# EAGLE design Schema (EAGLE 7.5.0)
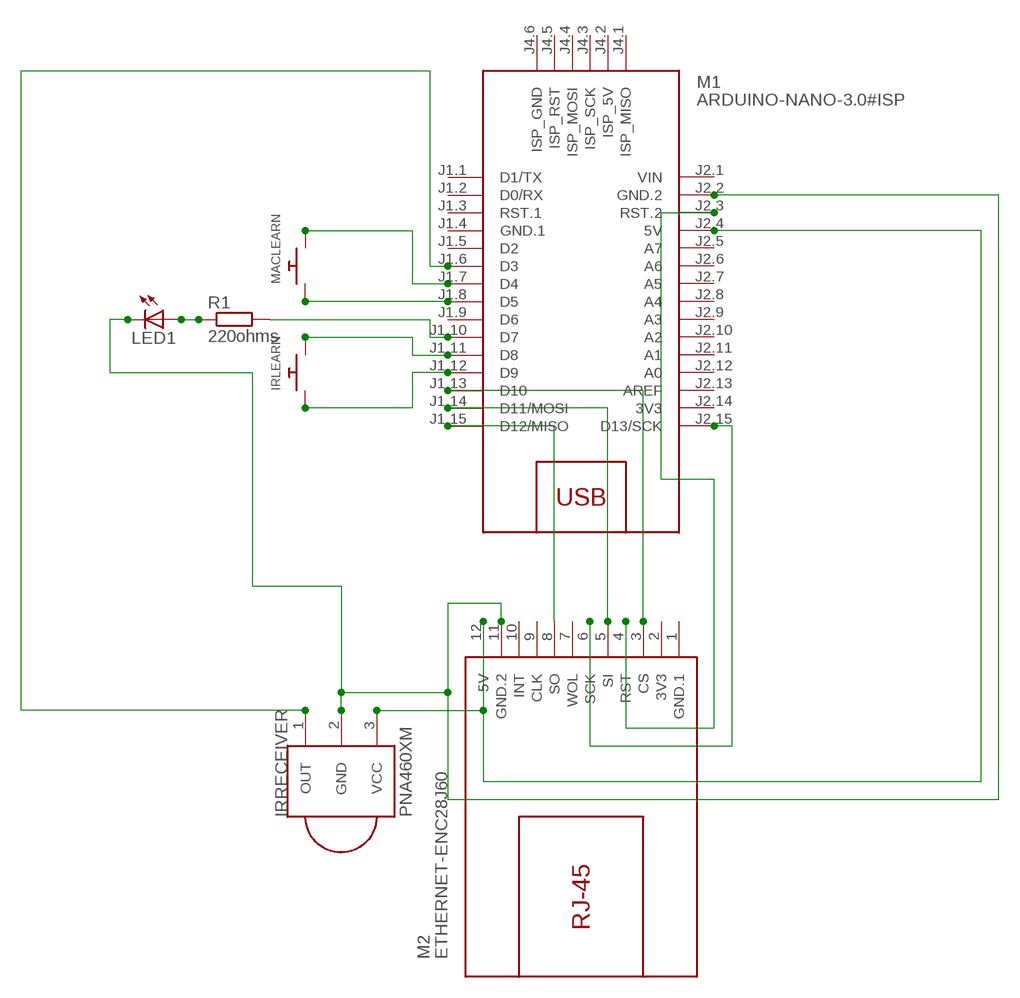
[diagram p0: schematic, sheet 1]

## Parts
IRLEARN  SWITCH_PUSHBUTTONEVQ-PE  [TACT_PANA-EVQ]
IRRECEIVER  PNA460XM  [PNA460XM]
LED1  LED5MM  [LED5MM]
M1  ARDUINO-NANO-3.0#ISP  [ARDUINO-NANO-3.0#ISP]
M2  ETHERNET-ENC28J60  [ETHERNET-ENC28J60]
MACLEARN  SWITCH_PUSHBUTTONEVQ-PE  [TACT_PANA-EVQ]
R1  220ohms  R-EU_0207/5V  [0207/5V]

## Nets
N$1: IRRECEIVER.2(GND) LED1.K(C) M1.J2.2(GND.2) M2.11(GND.2)
N$2: IRRECEIVER.3(VCC) M1.J2.4(5V) M2.12(5V)
N$3: M1.J1.13(D10) M2.3(CS)
N$4: M1.J2.3(RST.2) M2.4(RST)
N$5: M1.J1.14(D11/MOSI) M2.5(SI)
N$6: M1.J1.15(D12/MISO) M2.8(SO)
N$7: M1.J2.15(D13/SCK) M2.6(SCK)
N$8: LED1.A R1.1
N$9: IRRECEIVER.1(OUT) M1.J1.6(D3)
N$10: M1.J1.7(D4) MACLEARN.P$2
N$11: M1.J1.8(D5) MACLEARN.P$1
N$12: IRLEARN.P$2 M1.J1.11(D8)
N$13: IRLEARN.P$1 M1.J1.12(D9)
N$14: M1.J1.10(D7) R1.2
Unconnected: M1.J1.1(D1/TX) M1.J1.2(D0/RX) M1.J1.3(RST.1) M1.J1.5(D2) M1.J1.9(D6) M1.J2.5(A7) M1.J2.6(A6) M1.J2.7(A5) M1.J2.8(A4) M1.J2.9(A3) M1.J2.10(A2) M1.J2.11(A1) M1.J2.12(A0) M1.J2.13(AREF) M1.J4.1(ISP_MISO) M1.J4.2(ISP_5V) M1.J4.3(ISP_SCK) M1.J4.4(ISP_MOSI) M1.J4.5(ISP_RST) M1.J4.6(ISP_GND) M2.7(WOL) M2.9(CLK) M2.10(INT)

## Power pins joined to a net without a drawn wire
3V3: M1.J2.14(3V3) M2.2(3V3)
GND.1: M1.J1.4(GND.1) M2.1(GND.1)
VIN: M1.J2.1(VIN)

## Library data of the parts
IRLEARN MACLEARN = adafruit:SWITCH_PUSHBUTTON: Buttons
IRRECEIVER = adafruit:PNA460XM: IR 38KHz receiver PNA4602 and related receivers http://www.ladyada.net/library/pcb/eaglelibrary.html
LED1 = adafruit:LED: LED
M1 = diy-modules:ARDUINO-NANO-3.0#ISP: Arduino Nano 3.0 with ISP pads
M2 = diy-modules:ETHERNET-ENC28J60: Ethernet Module based on ENC28J60 chip
R1 = resistor:R-EU_: RESISTOR, European symbol

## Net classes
0 default: clearance 0.205 mm

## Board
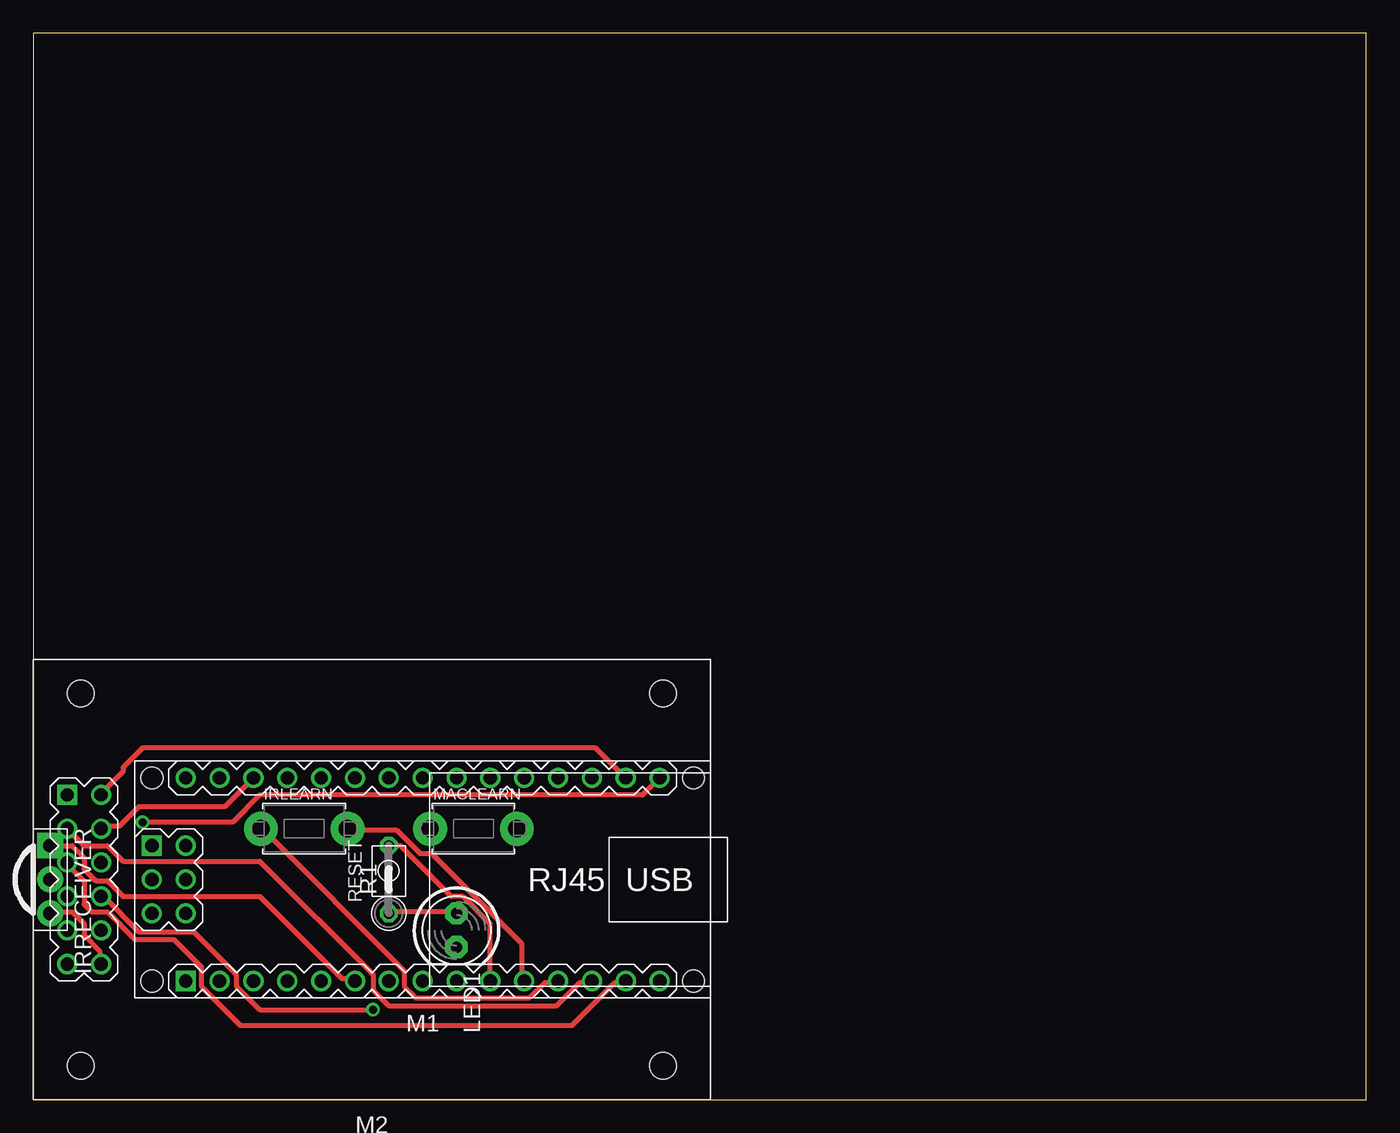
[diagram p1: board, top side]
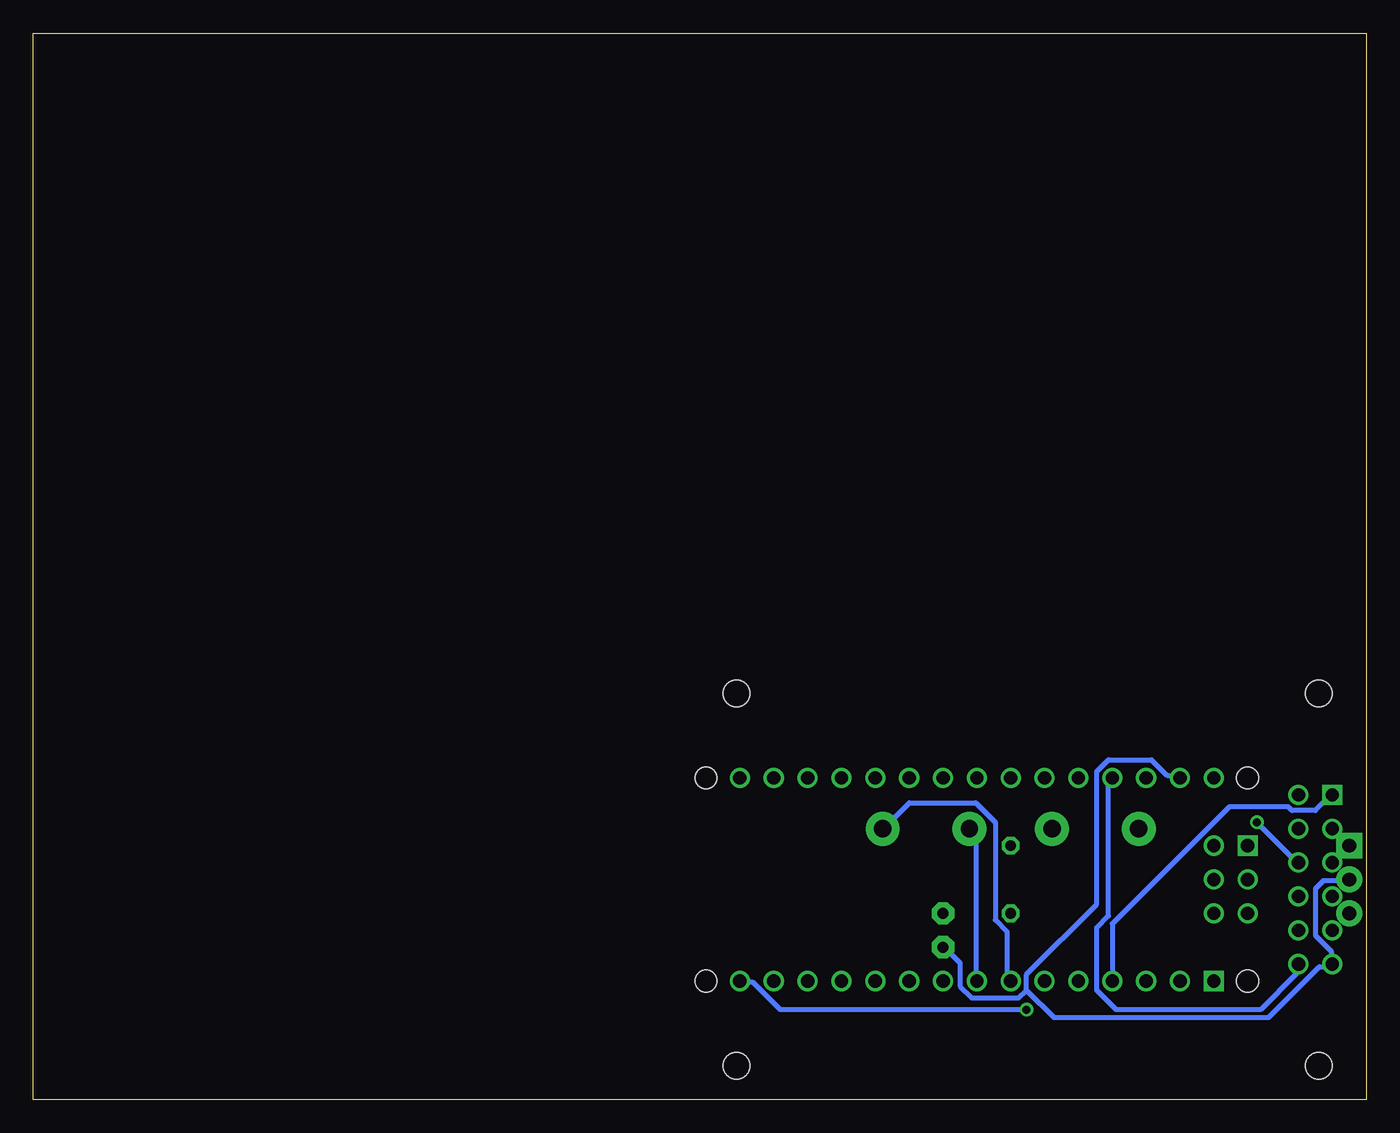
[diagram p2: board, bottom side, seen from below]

Size 100 x 80 mm. Coordinates in mm from the lower left corner, seen from the top.
Outline: 0,0 100,0 100,80 0,80 0,0
Copper layers (1*16): Top 0.035mm / dielectric 1.5mm / Bottom 0.035mm
Design rules "default *": minimum track width 15mil, minimum drill 24mil, track to track 8mil, track to pad 8mil, pad to pad 8mil, via to via 8mil, smd to smd 8mil, copper to edge 40mil, drill to drill 8mil, minimum pad ring 10mil, minimum via ring 8mil, stop-mask expansion 8mil, vias tented up to drill 0mil, thermal gap 10mil

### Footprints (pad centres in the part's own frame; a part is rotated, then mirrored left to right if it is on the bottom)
TACT_PANA-EVQ = drill 1.3 pad 2.54: P$1 -3.25,0; P$2 3.25,0
PNA460XM = drill 1.016 pad 1.93 square: 1 -2.54,0 | drill 1.016 pad 1.93: 2 0,0; 3 2.54,0
LED5MM = drill 0.813 pad 1.676 octagon: A -1.27,0; K 1.27,0
ARDUINO-NANO-3.0#ISP = drill 1 square: J1.1 17.78,7.62; J4.1 20.32,-2.54 | drill 1: J1.2 15.24,7.62; J1.3 12.7,7.62; J1.4 10.16,7.62; J1.5 7.62,7.62; J1.6 5.08,7.62; J1.7 2.54,7.62; J1.8 0,7.62; J1.9 -2.54,7.62; J1.10 -5.08,7.62; J1.11 -7.62,7.62; J1.12 -10.16,7.62; J1.13 -12.7,7.62; J1.14 -15.24,7.62; J1.15 -17.78,7.62; J2.1 17.78,-7.62; J2.2 15.24,-7.62; J2.3 12.7,-7.62; J2.4 10.16,-7.62; J2.5 7.62,-7.62; J2.6 5.08,-7.62; J2.7 2.54,-7.62; J2.8 0,-7.62; J2.9 -2.54,-7.62; J2.10 -5.08,-7.62; J2.11 -7.62,-7.62; J2.12 -10.16,-7.62; J2.13 -12.7,-7.62; J2.14 -15.24,-7.62; J2.15 -17.78,-7.62; J4.2 17.78,-2.54; J4.3 20.32,0; J4.4 17.78,0; J4.5 20.32,2.54; J4.6 17.78,2.54 | hole 1.651: -20.32,7.62; -20.32,-7.62; 20.32,-7.62; 20.32,7.62
ETHERNET-ENC28J60 = drill 1 square: 1 22.86,-6.35 | drill 1: 2 20.32,-6.35; 3 22.86,-3.81; 4 20.32,-3.81; 5 22.86,-1.27; 6 20.32,-1.27; 7 22.86,1.27; 8 20.32,1.27; 9 22.86,3.81; 10 20.32,3.81; 11 22.86,6.35; 12 20.32,6.35 | hole 2: -21.844,13.97; 21.844,13.97; -21.844,-13.97; 21.844,-13.97
0207/5V = drill 0.813 octagon: 1 -2.54,0; 2 2.54,0

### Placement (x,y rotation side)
IRLEARN  20.32,20.32 0 top
IRRECEIVER  1.27,16.51 270 top
LED1  31.75,12.7 270 top
M1  29.21,16.51 180 top
M2  25.4,16.51 180 top
MACLEARN  33.02,20.32 0 top
R1  26.67,16.51 90 top

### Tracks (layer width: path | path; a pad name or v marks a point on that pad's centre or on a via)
3V3
  Top 0.381: M2.2 5.27,23.15 6.74,24.61 6.74,24.91 8.2,26.37 42.19,26.37 44.24,24.32 M1.J2.14
GND.1
  Bottom 0.381: M1.J1.4 19.05,9.08 19.05,13.19 10.26,21.98 5.86,21.98 5.57,21.68 3.81,21.68 2.64,22.85 M2.1
N$1
  Bottom 0.381: IRRECEIVER.2 1.47,16.41 3.22,16.41 3.81,15.82 3.81,12.31 2.64,11.13 2.64,10.26 M2.11 2.64,9.96 3.52,9.96 7.33,6.15 23.44,6.15 25.49,8.2 | 25.49,8.2 25.49,9.38 20.22,14.65 20.22,24.61 19.34,25.49 16.11,25.49 14.94,24.32 14.06,24.32 M1.J2.2 | 25.49,8.2 26.08,7.62 29.59,7.62 30.47,8.5 30.47,10.26 31.64,11.43 LED1.K
N$2
  Top 0.381: M2.12 4.98,10.26 4.98,11.13 3.81,12.31 3.81,13.19 2.93,14.06 1.47,14.06 IRRECEIVER.3
  Bottom 0.381: M1.J2.4 19.34,24.03 19.34,13.77 20.22,12.89 20.22,8.2 18.75,6.74 7.91,6.74 5.27,9.38 5.27,9.96 M2.12
N$3
  Top 0.381: M1.J1.13 41.9,8.79 41.02,8.79 39.26,7.03 26.66,7.03 25.49,8.2 25.49,9.38 16.99,17.87 6.74,17.87 5.57,19.05 3.81,19.05 2.64,20.22 M2.3
N$4
  Top 0.381: M2.4 5.27,20.51 6.45,20.51 7.91,21.98 14.36,21.98 16.41,24.03 M1.J2.3
N$5
  Top 0.381: M1.J1.14 44.24,8.79 43.66,8.79 40.43,5.57 15.53,5.57 12.6,8.5 12.6,9.96 10.55,12.01 7.62,12.01 5.57,14.06 4.39,14.06 3.81,14.65 3.81,16.41 2.64,17.58 M2.5
N$6  (via drill 0.61)
  Top 0.381: v25.49,6.74 16.99,6.74 15.24,8.5 15.24,9.38 12.01,12.6 7.91,12.6 5.27,15.24 M2.8
  Bottom 0.381: v25.49,6.74 43.95,6.74 46,8.79 46.88,8.79 M1.J1.15
N$7  (via drill 0.61)
  Top 0.381: v8.2,20.8 14.94,20.8 16.99,22.85 45.71,22.85 46.88,24.03 M1.J2.15
  Bottom 0.381: v8.2,20.8 5.27,17.87 M2.6
N$8
  Top 0.381: R1.1 26.96,14.06 31.64,14.06 LED1.A
N$9
  Top 0.381: M1.J1.6 24.03,9.08 23.15,9.08 16.99,15.24 6.74,15.24 5.57,16.41 4.69,16.41 3.81,17.29 3.81,18.17 2.93,19.05 1.47,19.05 IRRECEIVER.1
N$10
  Bottom 0.381: M1.J1.7 26.96,9.08 26.96,12.6 27.84,13.48 27.84,20.8 29.3,22.27 34.28,22.27 36.04,20.51 MACLEARN.P$2
N$11
  Bottom 0.381: M1.J1.8 29.3,9.08 29.3,19.92 29.59,20.22 MACLEARN.P$1
N$12
  Top 0.381: M1.J1.11 36.62,9.08 36.62,11.72 29.89,18.46 29.01,18.46 27.25,20.22 23.73,20.22 IRLEARN.P$2
N$13
  Top 0.381: M1.J1.12 39.26,8.79 38.38,8.79 37.21,7.62 28.71,7.62 27.84,8.5 27.84,9.67 17.29,20.22 IRLEARN.P$1
N$14
  Top 0.381: R1.2 26.96,19.05 27.54,19.05 31.35,15.24 32.23,15.24 34.28,13.19 34.28,9.08 M1.J1.10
